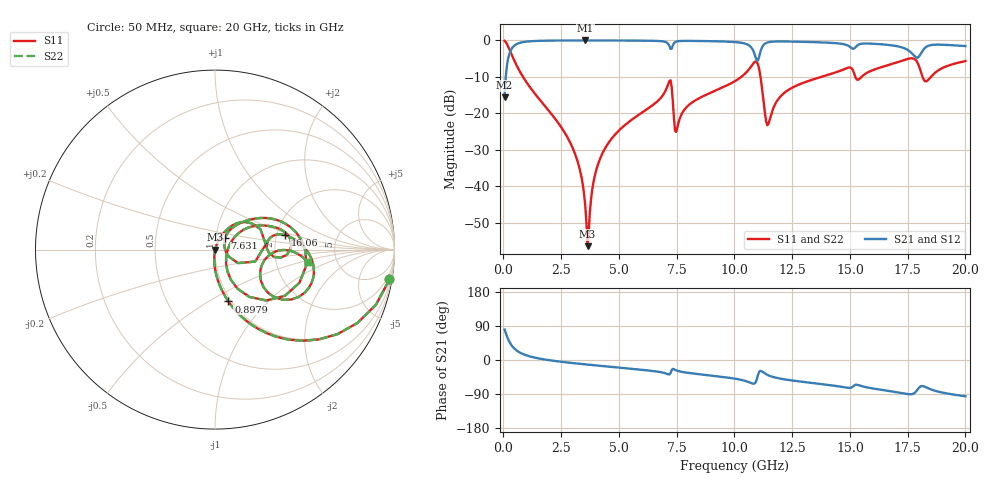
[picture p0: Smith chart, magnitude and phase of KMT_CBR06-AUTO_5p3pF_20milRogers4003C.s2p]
! Data measured by Modelithics Inc. support@modelithics.com 813-866-6335
! KEMET CBR06-AUTO 5.3pF, Pad Width= 0.851mm, Pad Length= 0.64mm, Pad Gap= 0.62mm, 20mil Rogers 4003C substrate Data, January 2022
# hz S ma R 50
! 2 Port Network Data from SP1.SP block
! freq  magS11  angS11  magS21  angS21  magS12  angS12  magS22  angS22
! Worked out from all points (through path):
!   401 points, 50 MHz to 20 GHz, reference 50 ohm
!   highest |S21| = -0.01 dB at 3.541 GHz (marker M1); lowest = -15.6 dB at 50 MHz (marker M2)
!   group delay of S21, straight-line fit = 15.2 ps
!   lowest |S11| = -56.4 dB at 3.641 GHz (marker M3), VSWR 1.00, Z = 50.1 - j0.0799 ohm
!   |S11| at or under -10 dB: 847.1 MHz to 10.29 GHz (9.447 GHz wide, 170 % of centre); 11.13 GHz to 13.76 GHz (2.628 GHz wide, 21.1 % of centre); 18.15 GHz to 18.51 GHz (359.8 MHz wide, 1.96 % of centre)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
!   |S22| runs from -56.4 to -0.1 dB; largest |S21 - S12| = 0
!   S11 on the Smith chart (normalised r, x): 50 MHz: 1, -12; 897.9 MHz: 0.97, -0.61; 7.631 GHz: 1.11, +0.14; 16.06 GHz: 2.23, +0.43; 20 GHz: 3.05, -0.58
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5e7  0.9862 -9.7  0.1656 80.3  0.1656 80.3  0.9862 -9.7
2.99375e8  0.7027 -46.3  0.7108 43.6  0.7108 43.6  0.7027 -46.3
8.97875e8  0.2982 -75.5  0.9537 14.3  0.9537 14.3  0.2982 -75.5
2.74325e9  0.04863 -94.9  0.9975 -6.4  0.9975 -6.4  0.04863 -94.9
3.391625e9  0.0127 -94.4  0.9984 -10.6  0.9984 -10.6  0.0127 -94.4
3.54125e9  0.005454 -86.6  0.9985 -11.6  0.9985 -11.6  0.005454 -86.6
3.641e9  0.001518 -31.7  0.9984 -12.2  0.9984 -12.2  0.001518 -31.7
3.990125e9  0.01552 70.2  0.9982 -14.2  0.9982 -14.2  0.01552 70.2
4.389125e9  0.03276 70.6  0.9977 -16.6  0.9977 -16.6  0.03276 70.6
6.73325e9  0.1535 56.0  0.9807 -31.3  0.9807 -31.3  0.1535 56.0
7.182125e9  0.2776 24.2  0.8403 -38.2  0.8403 -38.2  0.2776 24.2
7.481375e9  0.05578 22.1  0.9625 -27.3  0.9625 -27.3  0.05578 22.1
7.631e9  0.08454 48.8  0.98 -30.1  0.98 -30.1  0.08454 48.8
1.0025e10  0.2771 38.4  0.9489 -49.2  0.9489 -49.2  0.2771 38.4
1.097262e10  0.5054 -21.5  0.5269 -50.4  0.5269 -50.4  0.5054 -21.5
1.147138e10  0.07168 1.3  0.9451 -40.6  0.9451 -40.6  0.07168 1.3
1.336662e10  0.2894 27.7  0.9487 -60.7  0.9487 -60.7  0.2894 27.7
1.605988e10  0.3994 11.6  0.8982 -75.8  0.8982 -75.8  0.3994 11.6
1.670825e10  0.4641 5.4  0.8638 -81.9  0.8638 -81.9  0.4641 5.4
1.790525e10  0.5093 -33.0  0.579 -79.8  0.579 -79.8  0.5093 -33.0
1.830425e10  0.2751 -17.4  0.8152 -72.2  0.8152 -72.2  0.2751 -17.4
2e10  0.5207 -7.6  0.8363 -95.8  0.8363 -95.8  0.5207 -7.6
